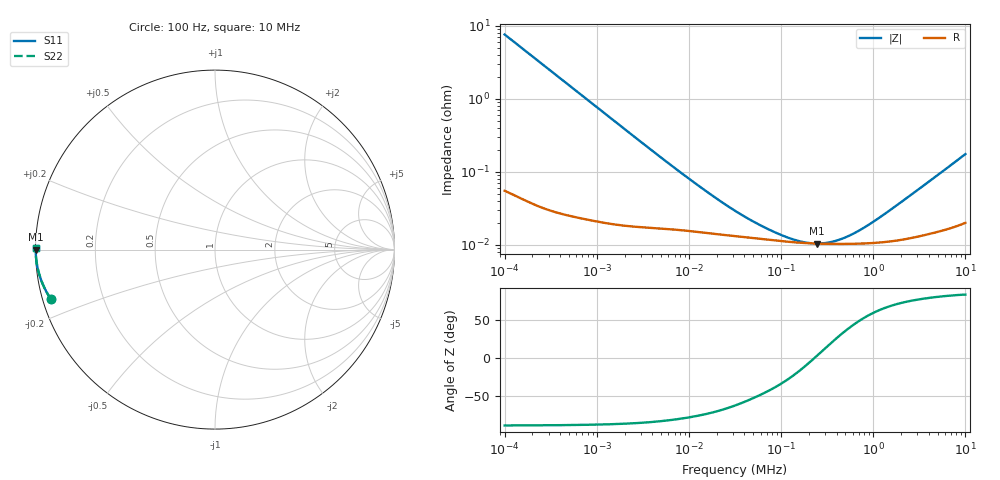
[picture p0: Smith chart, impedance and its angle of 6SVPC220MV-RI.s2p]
!  *** S-Parameter ***
!  Copyright (C) Panasonic Industry
!  Conductive Polymer Aluminum Solid Capacitors (OS-CON)
!  Parts No. 6SVPC220MV
! Touchstone file from project
# GHZ S RI R 50.000000
! Modal data exported
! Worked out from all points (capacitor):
!   401 points, 100 Hz to 10 MHz, reference 50 ohm
!   read as one part in shunt: C = 208 uF near 105.9 Hz
!   lowest |Z| = 10.4 mohm at 244.1 kHz (marker M1)
!   series resonance near 232.7 kHz, so ESL is about 2.2 nH
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1e-07  -0.9132 -0.278  0.0868 -0.278  0.0868 -0.278  -0.9132 -0.278
! Port Impedance 5.000000E+001 0.000000E+000 5.000000E+001 0.000000E+000
1.059254e-07  -0.9217 -0.265  0.0783 -0.265  0.0783 -0.265  -0.9217 -0.265
1.496236e-07  -0.9584 -0.1954  0.0416 -0.1954  0.0416 -0.1954  -0.9584 -0.1954
2.440619e-07  -0.9833 -0.1232  0.0167 -0.1232  0.0167 -0.1232  -0.9833 -0.1232
3.981072e-07  -0.993 -0.0764  0.00695 -0.0764  0.00695 -0.0764  -0.993 -0.0764
6.878599e-07  -0.9971 -0.0445  0.0029 -0.0445  0.0029 -0.0445  -0.9971 -0.0445
1.539927e-06  -0.9988 -0.02  0.00116 -0.02  0.00116 -0.02  -0.9988 -0.02
4.731513e-06  -0.9993 -0.00657  0.000716 -0.00657  0.000716 -0.00657  -0.9993 -0.00657
1.412538e-05  -0.9994 -0.00227  0.000596 -0.00227  0.000596 -0.00227  -0.9994 -0.00227
3.162278e-05  -0.9995 -0.00105  0.00053 -0.00105  0.00053 -0.00105  -0.9995 -0.00105
5.463865e-05  -0.9995 -0.000614  0.000492 -0.000614  0.000492 -0.000614  -0.9995 -0.000614
9.71628e-05  -0.9995 -0.000322  0.000453 -0.000322  0.000453 -0.000322  -0.9995 -0.000322
0.0001496236  -0.9996 -0.000154  0.000431 -0.000154  0.000431 -0.000154  -0.9996 -0.000154
0.0002175204  -0.9996 -2.32e-05  0.00042 -2.32e-05  0.00042 -2.32e-05  -0.9996 -2.32e-05
0.0002440619  -0.9996 1.65e-05  0.000417 1.65e-05  0.000417 1.65e-05  -0.9996 1.65e-05
0.0003548134  -0.9996 0.000152  0.000413 0.000152  0.000413 0.000152  -0.9996 0.000152
0.0004340103  -0.9996 0.000233  0.000413 0.000233  0.000413 0.000233  -0.9996 0.000233
0.0005308844  -0.9996 0.000323  0.000413 0.000323  0.000413 0.000323  -0.9996 0.000323
0.0008413951  -0.9996 0.000585  0.00042 0.000585  0.00042 0.000585  -0.9996 0.000585
0.001496236  -0.9996 0.00109  0.000446 0.00109  0.000446 0.00109  -0.9996 0.00109
0.009440609  -0.9992 0.00658  0.000822 0.00658  0.000822 0.00658  -0.9992 0.00658
0.01  -0.9991 0.00696  0.00085 0.00696  0.00085 0.00696  -0.9991 0.00696
